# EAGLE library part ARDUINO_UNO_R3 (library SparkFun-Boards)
Arduino R3 Footprint with SPI header Arduino Uno R3 Compatible Footprint. Matches PCB size of the original board. SparkFun Products: SAMD21 Dev Breakout RedBoard R3 Stackable Headers
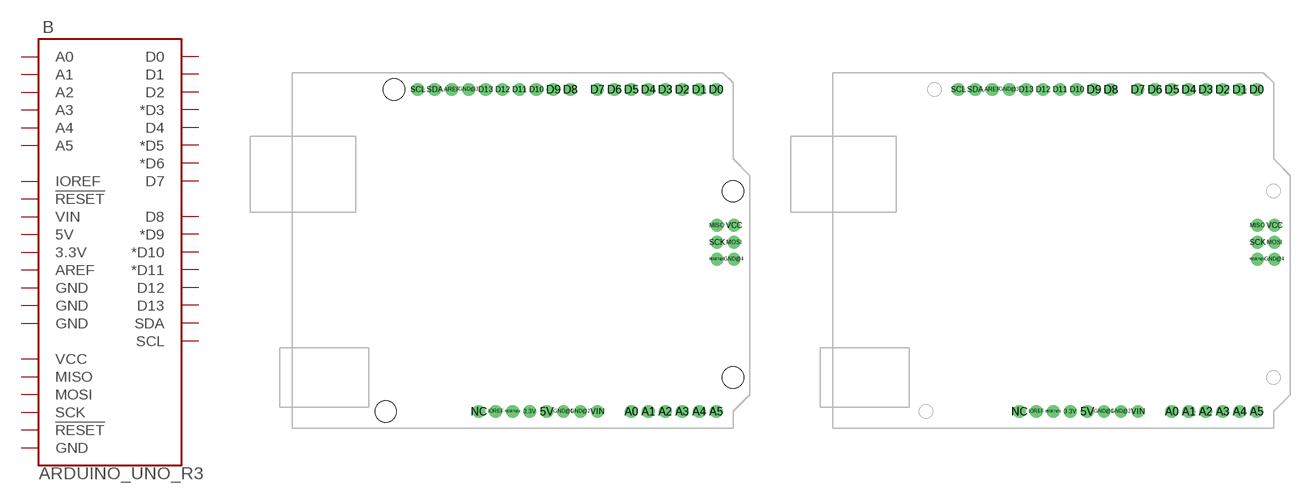
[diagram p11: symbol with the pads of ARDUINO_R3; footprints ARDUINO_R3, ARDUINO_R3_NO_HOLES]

Designator prefix B

## ARDUINO_UNO_R3  [ARDUINO_R3]
3.3V  3.3V
5V  5V
A0  A0
A1  A1
A2  A2
A3  A3
A4  A4
A5  A5
AREF  AREF
D0  D0
D1  D1
D2  D2
D3  *D3
D4  D4
D5  *D5
D6  *D6
D7  D7
D8  D8
D9  *D9
D10  *D10
D11  *D11
D12  D12
D13  D13
GND@1  GND
GND@2  GND
GND@3  GND
GND@4  GND
IOREF  IOREF
MISO  MISO
MOSI  MOSI
RESET@1  !RESET!
RESET@2  !RESET!
SCK  SCK
SCL  SCL
SDA  SDA
VCC  VCC
VIN  VIN

## ARDUINO_UNO_R3NO_HOLES  [ARDUINO_R3_NO_HOLES]
Pads as for ARDUINO_R3

## ARDUINO_UNO_R3LOCK_HOLES  [ARDUINO_R3_LOCK_HOLES]
Pads as for ARDUINO_R3

## Footprint ARDUINO_R3 (pad centres in mm)
Arduino Uno R3 Footprint Includes mounting holes, and holes for ICSP header Specifications: Pin count: 38 Area:2.7x2.1in Datasheet referenced for footprint: Example device(s): Arduino Uno R3
drill 1.016 pad 1.93: 3.3V 2.54,-24.13; 5V 5.08,-24.13; A0 17.78,-24.13; A1 20.32,-24.13; A2 22.86,-24.13; A3 25.4,-24.13; A4 27.94,-24.13; A5 30.48,-24.13; AREF -9.144,24.13; D0 30.48,24.13; D1 27.94,24.13; D2 25.4,24.13; D3 22.86,24.13; D4 20.32,24.13; D5 17.78,24.13; D6 15.24,24.13; D7 12.7,24.13; D8 8.636,24.13; D9 6.096,24.13; D10 3.556,24.13; D11 1.016,24.13; D12 -1.524,24.13; D13 -4.064,24.13; GND@1 7.62,-24.13; GND@2 10.16,-24.13; GND@3 -6.604,24.13; GND@4 33.16,-1.32; IOREF -2.54,-24.13; MISO 30.62,3.76; MOSI 33.16,1.22; NC -5.08,-24.13; RESET@1 0,-24.13; RESET@2 30.62,-1.32; SCK 30.62,1.22; SCL -14.224,24.13; SDA -11.684,24.13; VCC 33.16,3.76; VIN 12.7,-24.13
hole 3.175 at -17.78,24.13
hole 3.175 at 33.02,8.89
hole 3.175 at 33.02,-19.05
hole 3.175 at -19.05,-24.13

## Footprint ARDUINO_R3_NO_HOLES (pad centres in mm)
Arduino Uno R3 Footprint Includes holes for ICSP header Specifications: Pin count: 38 Area:2.7x2.1in Example device(s): Arduino Uno R3
drill 1.016 pad 1.93: 3.3V 1.27,-24.13; 5V 3.81,-24.13; A0 16.51,-24.13; A1 19.05,-24.13; A2 21.59,-24.13; A3 24.13,-24.13; A4 26.67,-24.13; A5 29.21,-24.13; AREF -10.414,24.13; D0 29.21,24.13; D1 26.67,24.13; D2 24.13,24.13; D3 21.59,24.13; D4 19.05,24.13; D5 16.51,24.13; D6 13.97,24.13; D7 11.43,24.13; D8 7.366,24.13; D9 4.826,24.13; D10 2.286,24.13; D11 -0.254,24.13; D12 -2.794,24.13; D13 -5.334,24.13; GND@1 6.35,-24.13; GND@2 8.89,-24.13; GND@3 -7.874,24.13; GND@4 31.89,-1.32; IOREF -3.81,-24.13; MISO 29.35,3.76; MOSI 31.89,1.22; NC -6.35,-24.13; RESET@1 -1.27,-24.13; RESET@2 29.35,-1.32; SCK 29.35,1.22; SCL -15.494,24.13; SDA -12.954,24.13; VCC 31.89,3.76; VIN 11.43,-24.13

## Footprint ARDUINO_R3_LOCK_HOLES (pad centres in mm)
drill 1.016 pad 1.93: 3.3V 35.56,2.667; 5V 38.1,2.413; A0 50.8,2.413; A1 53.34,2.667; A2 55.88,2.413; A3 58.42,2.667; A4 60.96,2.413; A5 63.5,2.667; AREF 23.876,50.927; D0 63.5,50.673; D1 60.96,50.927; D2 58.42,50.673; D3 55.88,50.927; D4 53.34,50.673; D5 50.8,50.927; D6 48.26,50.673; D7 45.72,50.927; D8 41.656,50.673; D9 39.116,50.927; D10 36.576,50.673; D11 34.036,50.927; D12 31.496,50.673; D13 28.956,50.927; GND@1 40.64,2.667; GND@2 43.18,2.413; GND@3 26.416,50.673; GND@4 66.18,25.223; IOREF 30.48,2.667; MISO 63.64,30.557; MOSI 66.18,27.89; NC 27.94,2.413; RESET@1 33.02,2.413; RESET@2 63.64,25.223; SCK 63.64,27.89; SCL 18.796,50.927; SDA 21.336,50.673; VCC 66.18,30.557; VIN 45.72,2.667
hole 3.175 at 15.24,50.8
hole 3.175 at 66.04,35.56
hole 3.175 at 66.04,7.62
hole 3.175 at 13.97,2.54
